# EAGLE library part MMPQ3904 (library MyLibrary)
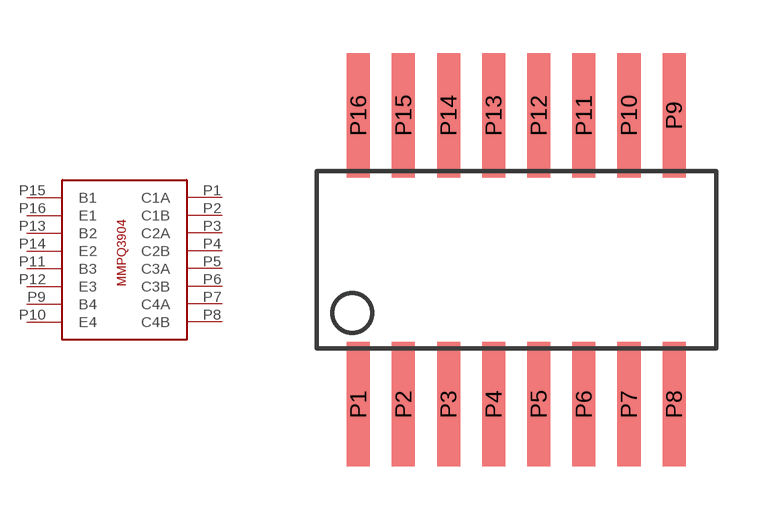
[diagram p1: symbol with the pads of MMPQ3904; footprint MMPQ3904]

Designator prefix -

## MMPQ3904  [MMPQ3904]
P1  C1A
P2  C1B
P3  C2A
P4  C2B
P5  C3A
P6  C3B
P7  C4A
P8  C4B
P9  B4
P10  E4
P11  B3
P12  E3
P13  B2
P14  E2
P15  B1
P16  E1

## Footprint MMPQ3904 (pad centres in mm)
smd 0.65 x 3.5: P1 -5.08,-4.07; P2 -3.81,-4.07; P3 -2.54,-4.07; P4 -1.27,-4.07; P5 0,-4.07; P6 1.27,-4.07; P7 2.54,-4.07; P8 3.81,-4.07; P9 3.81,4.07; P10 2.54,4.07; P11 1.27,4.07; P12 0,4.07; P13 -1.27,4.07; P14 -2.54,4.07; P15 -3.81,4.07; P16 -5.08,4.07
